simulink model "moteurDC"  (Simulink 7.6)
settings: Solver=ode23tb  StartTime=0.0  StopTime=N  FixedStep=0.0001  RelTol=1e-3
InitFcn:
  | clc, clear all, close all
  | N=0.02;
StopFcn:
  | close all
  | load vitesse_position.mat
  | plotyy(x(1,:),x(2,:),x(1,:),x(3,:))
  | %axis([0 N 0 12])
  | grid
  | title('Position et vitesse angulaires')
  | delete *.mat
libraries: fl_lib x4, nesl_utility x4, AppliMechanical_lib x1

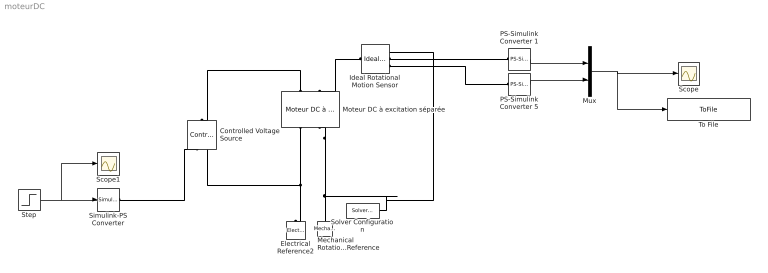
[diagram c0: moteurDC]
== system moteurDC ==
  Controlled Voltage Source : fl_lib/Electrical/Electrical Sources/Controlled Voltage Source  DialogController=NetworkEngine.DynNeDlgSource  SystemSampleTime=-1  i_Log=off  v_Log=off  LocalVarNames=|i|v  LocalVarDescs=|i|v  LocalVarLogging=[0 0]
  Electrical Reference2 : fl_lib/Electrical/Electrical Elements/Electrical Reference  DialogController=NetworkEngine.DynNeDlgSource  SystemSampleTime=-1  i_Log=off  LocalVarNames=|i  LocalVarDescs=|i  LocalVarLogging=[]
  Ideal Rotational Motion Sensor : fl_lib/Mechanical/Mechanical Sensors/Ideal Rotational Motion Sensor  DialogController=NetworkEngine.DynNeDlgSource  SystemSampleTime=-1  offset=0 rad  w_Log=off  t_Log=off  phi_Log=off  LocalVarNames=|w|t|phi  LocalVarDescs=|w|t|phi  LocalVarLogging=[0 0 0]
  Mechanical Rotational Reference : fl_lib/Mechanical/Rotational Elements/Mechanical Rotational Reference  DialogController=NetworkEngine.DynNeDlgSource  SystemSampleTime=-1  t_Log=off  LocalVarNames=|t  LocalVarDescs=|t  LocalVarLogging=[]
  Moteur DC à excitation séparée : AppliMechanical_lib/Moteur DC à excitation séparée  DialogController=NetworkEngine.DynNeDlgSource  SystemSampleTime=-1  K=0.1 N*m/A  Ri=4.9 Ohm  Li=1e-5 H  fr=0.02 N*m/(rad/s)  J=1e-5 kg*m^2  w_Log=off  i_Log=off  v_Log=off  t_Log=off  LocalVarNames=|w|i|v|t  LocalVarDescs=|w|i|v|t  LocalVarLogging=[0 0 0 0]
  Mux : Mux  Inputs=2
  PS-Simulink Converter 1 : nesl_utility/PS-Simulink Converter  DialogController=NetworkEngine.DynNeUtilDlgSource  SystemSampleTime=-1  PhysicalDomain=network_engine_domain  LeftPortType=input  RightPortType=output  SubClassName=ps_output  Unit=rad/s  AffineConversion=off
  PS-Simulink Converter 5 : nesl_utility/PS-Simulink Converter  DialogController=NetworkEngine.DynNeUtilDlgSource  SystemSampleTime=-1  PhysicalDomain=network_engine_domain  LeftPortType=input  RightPortType=output  SubClassName=ps_output  Unit=rad  AffineConversion=off
  Scope : Scope
  Scope1 : Scope
  Simulink-PS Converter : nesl_utility/Simulink-PS Converter  DialogController=NetworkEngine.DynNeUtilDlgSource  SystemSampleTime=-1  PhysicalDomain=network_engine_domain  LeftPortType=input  RightPortType=output  SubClassName=ps_input  Unit=1  AffineConversion=off  InputFilterTimeConstant=.001  UdotUserProvided=0
  Solver Configuration : nesl_utility/Solver Configuration  DialogController=NetworkEngine.DynNeUtilDlgSource  SystemSampleTime=-1  PhysicalDomain=network_engine_domain  LeftPortType=input  RightPortType=generic  SubClassName=solver  Accelerate=off  Profile=off  ResidualTolerance=1e-9  MaxNonlinIter=12  MaxModeIter=2  DoFixedCost=off  UseLocalSampling=off  DoDC=off  LinearAlgebra=Sparse  LocalSolverSampleTime=.001  LocalSolverChoice=NE_BACKWARD_EULER_ADVANCER  UseLocalSolver=off
  Step : Step  Time=0.005  After=12  SampleTime=0
  To File : ToFile  Filename=vitesse_position  MatrixName=x
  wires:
  Step/1 -> Simulink-PS Converter/1, Scope1/1
  PS-Simulink Converter 5/1 -> Mux/2
  Mux/1 -> To File/1, Scope/1
  PS-Simulink Converter 1/1 -> Mux/1
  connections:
  Simulink-PS Converter/RConn1 -- Controlled Voltage Source/RConn1
  Moteur DC à excitation séparée/LConn1 -- Controlled Voltage Source/LConn1
  Moteur DC à excitation séparée/RConn1 -- Electrical Reference2/LConn1 -- Controlled Voltage Source/RConn2
  Moteur DC à excitation séparée/RConn2 -- Mechanical Rotational Reference/LConn1 -- Ideal Rotational Motion Sensor/RConn1 -- Solver Configuration/RConn1
  Ideal Rotational Motion Sensor/LConn1 -- Moteur DC à excitation séparée/LConn2
  Ideal Rotational Motion Sensor/RConn2 -- PS-Simulink Converter 1/LConn1
  Ideal Rotational Motion Sensor/RConn3 -- PS-Simulink Converter 5/LConn1
